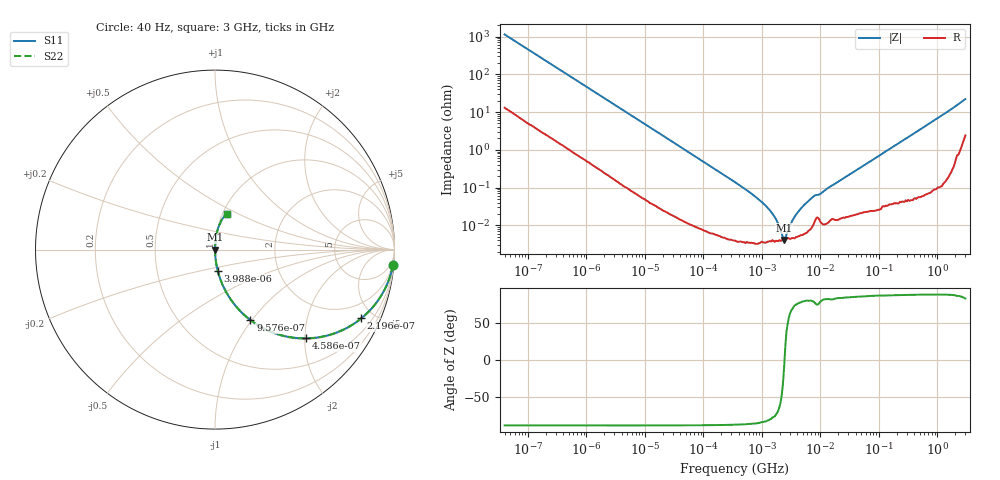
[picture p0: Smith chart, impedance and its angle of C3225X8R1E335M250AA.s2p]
! S-parameter Generated by TDK Corporation
! Copyright(C) 2015 TDK Corporation.
! All Rights Reserved.
! TDK P/N: C3225X8R1E335M250AA (Multilayer Ceramic Chip Capacitors)
! Property: C=3.3uF
! Size(LxWxT): 3.2x2.5x2.5mm, 0.126x0.098x0.098inches
! Model Type: s2p (Touchstone File Format Version 1.0)
! Frequency: DC=Yes Start=0.00004MHz Stop=3000MHz 396points Log-sweep
! Note: This model was converted from impedance.
! Model Generated on Jun. 23, 2015
! Hash(MD5):
! Port Assignments:
!  1 ---| |--- 2
! Applicable Conditions:
!  Temperature = 25 degC
!  DC Bias Voltage = 0 V
!  Small Signal Operation
! Terms and conditions regarding TDK Simulation Models
! (1)This simulation model is being provided solely for informational purposes. Please refer to the specifications of the products in terms of detailed characteristics of such products.
! (2)In no event shall TDK Corporation of any of its subsidiaries be liable for any loss or damage arising, directly or indirectly,
!  From any information contained in this simulation model, including, but not limited to loss or damages arising from any inaccuracies, omissions or errors in connection with such information.
! (3)Any and all copyrights on this simulation model are owned by TDK Corporation.
!  Duplication or redistribution of this simulation model without prior written permission from TDK Corporation is prohibited.
! (4)This simulation model is subject to any modification or change without any prior notice.
! (5)Neither TDK Corporation nor any of its subsidiaries shall make any warranty, express or implied,
!  Including but not limited to the correctness, implied warranties of merchantability and fitness for a particular purpose with respect to this simulation models.
! (6)The use of this simulation model shall be deemed to have consented to the terms and conditions hereof.
# MHz S MA R 50
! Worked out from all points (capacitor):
!   395 points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, 40 Hz to 3 GHz, reference 50 ohm
!   read as one part in series: C = 3.48 uF near 41.88 Hz
!   lowest |Z| = 4.07 mohm at 2.394 MHz (marker M1)
!   series resonance near 2.432 MHz, so ESL is about 1.2 nH
!   S11 on the Smith chart (normalised r, x): 40 Hz: 1, -23; 219.6 Hz: 1.05, -4.23; 458.6 Hz: 1.02, -2.04; 957.6 Hz: 1.01, -0.98; 3.988 kHz: 1.00, -0.24; 3 GHz: 1.05, +0.44
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4e-05  0.9952 -5.0  0.08741 84.3  0.08741 84.3  0.9952 -5.0
0.0001100992  0.9703 -13.4  0.2313 76.0  0.2313 76.0  0.9703 -13.4
0.0002195817  0.9003 -25.2  0.4256 64.2  0.4256 64.2  0.9003 -25.2
0.0004585594  0.7099 -44.2  0.6966 45.2  0.6966 45.2  0.7099 -44.2
0.000834128  0.4883 -60.2  0.8675 29.2  0.8675 29.2  0.4883 -60.2
0.0009576241  0.4388 -63.4  0.8939 26.0  0.8939 26.0  0.4388 -63.4
0.001741936  0.2612 -74.3  0.9625 15.1  0.9625 15.1  0.2612 -74.3
0.003988472  0.1184 -82.6  0.9918 6.8  0.9918 6.8  0.1184 -82.6
0.01739424  0.02767 -87.8  0.9993 1.6  0.9993 1.6  0.02767 -87.8
0.3464102  0.001391 -88.3  1 0.1  1 0.1  0.001391 -88.3
0.7574911  0.0005895 -86.8  1 0.0  1 0.0  0.0005895 -86.8
1.146211  0.0003356 -84.0  1 0.0  1 0.0  0.0003356 -84.0
1.510739  0.0002044 -78.6  1 0.0  1 0.0  0.0002044 -78.6
1.991197  9.308e-05 -64.2  1 0.0  1 0.0  9.308e-05 -64.2
2.393669  4.067e-05 -10.2  1 0.0  1 0.0  4.067e-05 -10.2
3.013016  9.728e-05 63.3  1 -0.0  1 -0.0  9.728e-05 63.3
4.15828  0.0002286 77.0  0.9999 -0.0  0.9999 -0.0  0.0002286 77.0
7.22376  0.000541 80.3  0.9999 -0.0  0.9999 -0.0  0.000541 80.3
9.969551  0.0006821 79.5  0.9999 -0.0  0.9999 -0.0  0.0006821 79.5
150.6385  0.01043 87.4  0.9996 -0.6  0.9996 -0.6  0.01043 87.4
949.3681  0.06455 85.5  0.997 -3.7  0.997 -3.7  0.06455 85.5
3000  0.2107 71.6  0.9548 -12.1  0.9548 -12.1  0.2107 71.6
